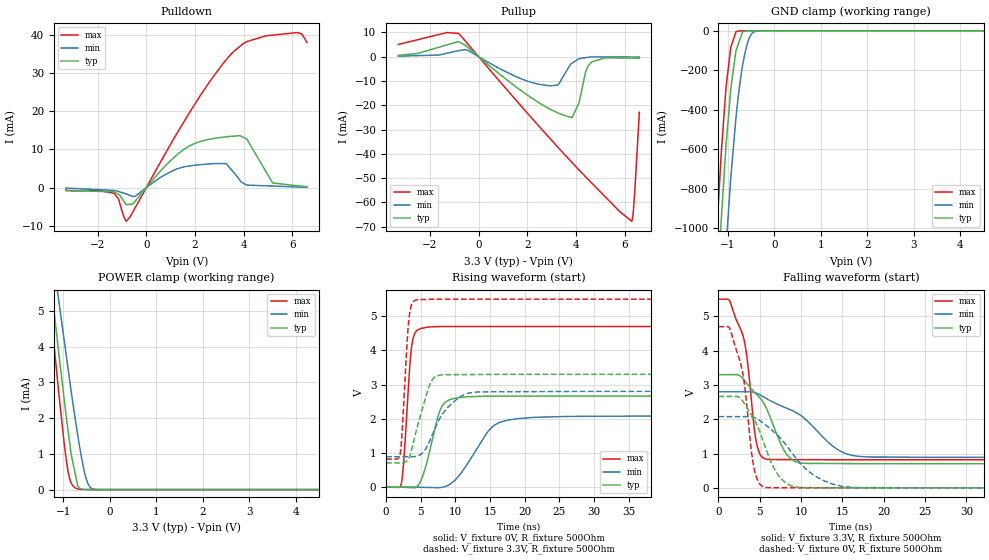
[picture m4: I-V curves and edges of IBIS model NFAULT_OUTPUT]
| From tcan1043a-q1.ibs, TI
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|   NFAULT_OUTPUT Model
[Model]   NFAULT_OUTPUT
Model_type   3-state
Polarity   Non-Inverting
Vmeas = 1.5
Vref = 0
Cref = 15pF
Rref = 100000
|   typ   min   max
C_comp   1.806pF   1.606pF   1.880pF
|  Where Nom  PVT is Nominal Process,   3.3V,  27C
|   Fast PVT is Strong Process,   5.5V, -55C
|   Slow PVT is Weak Process,   2.8V, 150C
[Voltage Range]   3.3   2.8   5.5
|Junction Temperature
[Temperature Range]   27   150   -55
[Pullup Reference]   3.3   2.8   5.5
[Pulldown Reference]   0   0   0
[Power Clamp Reference]   3.3   2.8   5.5
[GND Clamp Reference]   0   0   0
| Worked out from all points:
|   slope of the pulldown table from 0 to 0.495 V, typ, clamps not added: 133 ohm
|   slope of the pullup table from 0 to 0.495 V, typ, clamps not added: 119 ohm
|   GND clamp passes 1 mA (typ) near -0.62 V on its own axis
|   POWER clamp passes 1 mA (typ) near -0.83 V on its own axis
|   falling waveform, V_fixture 3.3V, R_fixture 500Ohm: 20-80 % time 3.27ns typ, 6.23ns min, 1.54ns max; typ from 3.3 V to 0.705 V
|   rising waveform, V_fixture 0V, R_fixture 500Ohm: 20-80 % time 1.97ns typ, 4.01ns min, 896ps max; typ from 0 V to 2.67 V
|   rising waveform, V_fixture 3.3V, R_fixture 500Ohm: 20-80 % time 2.1ns typ, 3.25ns min, 793ps max; typ from 0.705 V to 3.3 V
|   falling waveform, V_fixture 0V, R_fixture 500Ohm: 20-80 % time 2.82ns typ, 4.72ns min, 1.54ns max; typ from 2.67 V to 0 V
[Pulldown]
|   Voltage   I(typ)   I(min)   I(max)
-3.3V     -223.4uA   -100.9uA   -314.6uA
-1.331V   -1.084mA   -717.4uA   -1.468mA
-1.144V   -1.727mA   -994uA     -2.847mA
-825mV    -4.459mA   -1.616mA   -8.791mA
-451.1mV  -3.534mA   -2.217mA   -5.214mA
1.579V    10.15mA    5.487mA    17.57mA
3.276V    13.27mA    6.275mA    33.37mA
3.559V    13.45mA    4.229mA    35.43mA
4.124V    12.75mA    676.1uA    38.16mA
5.188V    1.221mA    425.8uA    39.88mA
6.211V    494.2uA    186.3uA    40.54mA
6.6V      218uA      95.24uA    37.93mA
[GND Clamp]
|   Voltage   I(typ)   I(min)   I(max)
-3.3V     -11.12A    -11.52A    -10.9A
-1.282V   -1.546A    -2.086A    -1.205A
-1.212V   -1.245A    -1.78A     -912.9mA
-1.141V   -957.4mA   -1.496A    -618.8mA
-1.037V   -578.9mA   -1.095A    -283.2mA
-935.2mV  -294.4mA   -742.9mA   -83mA
-825mV    -101.1mA   -440.8mA   -4.829mA
-731.1mV  -37.76mA   -250.3mA   -627.5uA
-635.8mV  -2.173mA   -117mA     -100.4uA
-534.2mV  -437.2uA   -33.87mA   -36.42uA
-427.3mV  -89.14uA   -3.563mA   -22.26uA
6.6V      0A         0A         0A
[Pullup]
|   Voltage   I(typ)   I(min)   I(max)
-3.3V     517.3uA    199.3uA    5.008mA
-825mV    6.2mA      2.45mA     9.568mA
2.852V    -21.16mA   -11.92mA   -32.79mA
3.263V    -23.19mA   -11.66mA   -37.34mA
3.841V    -25.06mA   -2.664mA   -43.63mA
4.124V    -18.99mA   -813.8uA   -46.67mA
4.393V    -6.283mA   -424.8uA   -49.41mA
4.643V    -2.171mA   -93.06uA   -51.97mA
6.289V    -606.9uA   -170.6uA   -67.74mA
6.338V    -610.8uA   -172.9uA   -65.52mA
6.41V     -616.5uA   -176.3uA   -55.86mA
6.6V      -631.7uA   -185.2uA   -22.96mA
[POWER Clamp]
|   Voltage   I(typ)   I(min)   I(max)
-3.3V     30.62mA    27.79mA    33.75mA
-1.495V   8.536mA    9.272mA    8.139mA
-1.276V   5.935mA    7.082mA    5.116mA
-1.25V    5.622mA    6.819mA    4.768mA
-1.093V   3.813mA    5.281mA    2.691mA
-930.6mV  2.014mA    3.732mA    809.6uA
-861.1mV  1.322mA    3.07mA     308.5uA
-730.4mV  382.1uA    1.891mA    39.47uA
-683.4mV  92.63uA    1.498mA    17.01uA
-511.4mV  3.93uA     332.1uA    1.313uA
-308.5mV  3.372nA    5.041uA    255.7nA
6.6V      0A         0A         0A
[Ramp]
R_load = 500
|   typ   min   max
dV/dt_r   1.5992/1.96395e-09   1.24612/4.00502e-09   2.81983/8.96134e-10
dV/dt_f   1.55682/3.2658e-09   1.14676/6.22643e-09   2.80844/1.53412e-09
[Falling Waveform]
V_fixture = 3.3V
V_fixture_min = 2.8V
V_fixture_max = 5.5V
R_fixture = 500Ohm
C_fixture = 0F
|   Time   V(typ)   V(min)   V(max)
0s        3.3V       2.8V       5.5V
1.304ns   3.301V     2.8V       5.473V
2.965ns   3.178V     2.801V     4.435V
3.506ns   3.017V     2.801V     3.686V
4.594ns   2.727V     2.759V     1.321V
5.961ns   2.229V     2.582V     827.4mV
9.203ns   776.3mV    2.219V     823.1mV
14.55ns   709.1mV    1.096V     819.5mV
18.05ns   705.6mV    901.5mV    819.5mV
200ns     705.3mV    888.7mV    819.3mV
[Rising Waveform]
V_fixture = 0V
V_fixture_min = 0V
V_fixture_max = 0V
R_fixture = 500Ohm
C_fixture = 0F
|   Time   V(typ)   V(min)   V(max)
0s        127.8pV    202.2nV    82.52pV
2.149ns   -722.7uV   -407.6uV   68.23mV
2.566ns   -4.662mV   -486.8uV   837.5mV
3.743ns   -19.11mV   -710.2uV   4.196V
5.961ns   793.9mV    -10.52mV   4.68V
7.504ns   2.08V      -18.44mV   4.697V
8.603ns   2.497V     22.85mV    4.698V
15.45ns   2.662V     1.785V     4.699V
21.45ns   2.665V     2.041V     4.699V
200ns     2.665V     2.077V     4.7V
[Rising Waveform]
V_fixture = 3.3V
V_fixture_min = 2.8V
V_fixture_max = 5.5V
R_fixture = 500Ohm
C_fixture = 0F
|   Time   V(typ)   V(min)   V(max)
0s        705.3mV    888.7mV    819.3mV
2.024ns   707.1mV    888.3mV    977.4mV
2.257ns   707.4mV    888.3mV    1.478V
3.29ns    848.7mV    888.1mV    4.924V
3.743ns   1.146V     888mV      5.376V
4.511ns   1.78V      907.5mV    5.482V
7.05ns    3.224V     1.718V     5.498V
10.25ns   3.29V      2.579V     5.5V
13.35ns   3.294V     2.785V     5.5V
200ns     3.3V       2.8V       5.5V
[Falling Waveform]
|Gnd
V_fixture = 0V
V_fixture_min = 0V
V_fixture_max = 0V
R_fixture = 500Ohm
C_fixture = 0F
|   Time   V(typ)   V(min)   V(max)
0s        2.665V     2.077V     4.7V
1.304ns   2.665V     2.077V     4.671V
2.566ns   2.625V     2.077V     3.721V
3.127ns   2.457V     2.077V     3.029V
4.31ns    2.002V     2.051V     561.3mV
5.861ns   1.06V      1.804V     8.195mV
8.503ns   91.49mV    1.145V     4.561mV
11.55ns   5.735mV    367.7mV    2.539mV
16.45ns   1.405mV    9.749mV    204.6uV
200ns     127.8pV    202.2nV    82.52pV
